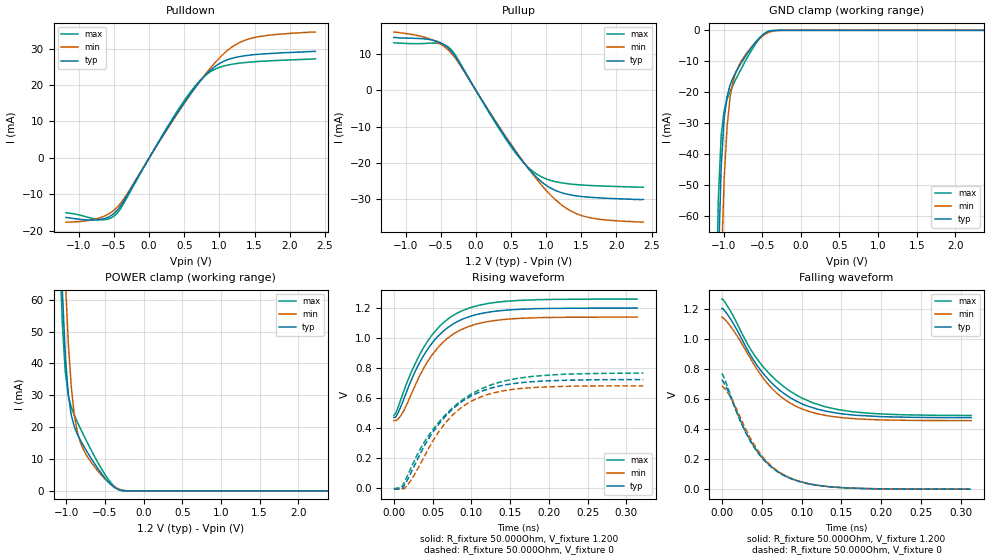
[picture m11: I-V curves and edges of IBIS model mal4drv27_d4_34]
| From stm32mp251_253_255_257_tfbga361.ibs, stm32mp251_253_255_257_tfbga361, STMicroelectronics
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[Model] mal4drv27_d4_34
Model_type   I/O
Polarity   Non-Inverting
Enable   Active-High
C_comp   1.656pF   1.652pF   1.661pF
C_comp_pullup   829.373fF   822.555fF   836.725fF
C_comp_pulldown 737.416fF   735.607fF   748.448fF
Vinh = 852.000mV
Vinl = 737.000mV
Vmeas = 795.000mV
Vref = 1.200V
Rref = 50Ohms
Cref = 0pF
[Model Spec]
Vinh   852.000mV   812.000mV   892.000mV
Vinl   737.000mV   697.000mV   777.000mV
Vmeas   795.000mV   755.000mV   834.000mV
Vref   1.200V   1.140V   1.260V
D_overshoot_ampl_h 0.24 NA   NA
D_overshoot_ampl_l 0.24 NA   NA
D_overshoot_area_l 300.000m NA   NA
D_overshoot_area_h 300.000m NA   NA
[Receiver Thresholds]
Vth = 795.000mV
Vth_min = 755.000mV
Vth_max = 834.000mV
Vinh_ac = 68.000mV
Vinh_dc = 68.000mV
Vinl_ac = -68.000mV
Vinl_dc = -68.000mV
Tslew_ac = 5.000ns
Threshold_sensitivity = 0.5
Reference_supply Pullup_ref
[Temperature Range]   25.000   125.000   -40.000
[Voltage Range]   1.200V   1.140V   1.260V
[GND Clamp Reference]   0.00V   0.00V   0.00V
[C Comp Corner]
| variable   typ   min   max
C_comp 1.661pF   1.656pF   1.652pF
C_comp_pullup 829.373fF   836.725fF   822.555fF
C_comp_pulldown 735.607fF   748.448fF   737.416fF
[Pulldown Reference]   0.00V   0.00V   0.00V
[POWER Clamp Reference]   1.200V   1.140V   1.260V
[Pullup Reference]   1.200V   1.140V   1.260V
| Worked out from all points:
|   slope of the pulldown table from 0 to 0.18 V, typ, clamps not added: 31.5 ohm
|   slope of the pullup table from 0 to 0.18 V, typ, clamps not added: 31.8 ohm
|   GND clamp passes 1 mA (typ) near -0.47 V on its own axis
|   POWER clamp passes 1 mA (typ) near -0.37 V on its own axis
|   rising waveform, R_fixture 50.000Ohm, V_fixture 1.200: 20-80 % time 51.2ps typ, 50.7ps min, 52.2ps max; typ from 0.472 V to 1.2 V
|   rising waveform, R_fixture 50.000Ohm, V_fixture 0: 20-80 % time 62.5ps typ, 57.9ps min, 71.8ps max; typ from -0.006 V to 0.724 V
|   falling waveform, R_fixture 50.000Ohm, V_fixture 1.200: 20-80 % time 62.9ps typ, 58.9ps min, 69.2ps max; typ from 1.2 V to 0.475 V
|   falling waveform, R_fixture 50.000Ohm, V_fixture 0: 20-80 % time 49.1ps typ, 48.9ps min, 49.5ps max; typ from 0.727 V to 0 V
[GND Clamp]
-1.184V   -313.6mA   -372.3mA   -285.9mA
-1.107V   -133mA     -190.9mA   -103.4mA
-1.069V   -76.66mA   -125mA     -55.43mA
-1.031V   -44.19mA   -77.99mA   -34.02mA
-992.7mV  -28.51mA   -48.19mA   -25.88mA
-954.6mV  -21.35mA   -31.1mA    -22.21mA
-916.4mV  -17.7mA    -21.78mA   -19.79mA
-878.2mV  -15.35mA   -16.61mA   -17.73mA
-801.8mV  -11.82mA   -11.34mA   -13.9mA
-610.9mV  -4.628mA   -4.618mA   -5.371mA
-458.2mV  -822.8uA   -1.198mA   -809uA
2.367V    18.95nA    454.6nA    6.243nA
[Power Clamp]
-1.167V   171.5mA    206.4mA    156.1mA
-1.091V   92.44mA    126.6mA    77.99mA
-1.053V   63.02mA    93.75mA    52.4mA
-1.015V   42.49mA    66.9mA     37.37mA
-976.4mV  30.34mA    46.72mA    30.02mA
-938.2mV  23.88mA    32.9mA     26.3mA
-900mV    20.31mA    24.15mA    23.84mA
-823.6mV  16.11mA    15.49mA    19.79mA
-747.3mV  12.87mA    11.46mA    16.02mA
-518.2mV  4.545mA    4.187mA    5.836mA
-365.4mV  856.5uA    1.078mA    1.107mA
2.384V    -12.74nA   -415.5nA   -4.625nA
[Pulldown]
-1.184V   -16.3mA    -17.6mA    -15mA
-725.5mV  -16.94mA   -16.55mA   -16.87mA
-572.7mV  -16.13mA   -15.3mA    -16.68mA
-458.2mV  -14.43mA   -13.55mA   -15.2mA
-305.5mV  -9.986mA   -9.58mA    -10.51mA
420mV     12.95mA    12.68mA    13.44mA
687.3mV   20.12mA    20.08mA    20.48mA
878.2mV   24.14mA    24.8mA     23.72mA
1.145V    27.12mA    29.93mA    25.57mA
1.375V    28.05mA    32.33mA    26.17mA
1.756V    28.67mA    33.75mA    26.66mA
2.367V    29.2mA     34.5mA     27.18mA
[Pullup]
-1.167V   14.6mA     16.1mA     13.16mA
-594.5mV  13.79mA    13.71mA    13.07mA
-480mV    12.94mA    12.49mA    12.8mA
-365.4mV  11.21mA    10.59mA    11.52mA
-250.9mV  8.092mA    7.721mA    8.443mA
283.6mV   -8.835mA   -8.586mA   -9.154mA
550.9mV   -16.57mA   -16.29mA   -16.91mA
780mV     -22.29mA   -22.41mA   -21.87mA
1.009V    -26.32mA   -27.79mA   -24.51mA
1.276V    -28.56mA   -32.42mA   -25.69mA
1.505V    -29.32mA   -34.57mA   -26.12mA
2.384V    -30.1mA    -36.4mA    -26.74mA
[Ramp]
R_load=50.000Ohm
dV/dt_r   434.850mV/58.000ps  410.159mV/55.500ps  461.550mV/63.000ps
dV/dt_f   434.850mV/57.000ps  410.159mV/55.000ps  461.550mV/61.000ps
[Rising waveform]
R_fixture=50.000Ohm
V_fixture=1.200
V_fixture_min=1.140
V_fixture_max=1.260
0s        472.2mV    451.1mV    485.7mV
4ps       488.5mV    455.5mV    521.4mV
12ps      584.3mV    509.5mV    637.6mV
27ps      773.4mV    680.4mV    825.2mV
41ps      906.4mV    822.7mV    959.8mV
62ps      1.038V     965.3mV    1.094V
85ps      1.118V     1.051V     1.175V
113ps     1.164V     1.102V     1.222V
153ps     1.189V     1.129V     1.248V
314ps     1.2V       1.14V      1.26V
[Rising waveform]
R_fixture=50.000Ohm
V_fixture=0
0s        -6.059mV   -4.191mV   -2.794mV
10ps      -6.059mV   -4.191mV   6.233mV
19ps      70.79mV    30.63mV    100.5mV
38ps      270mV      200.4mV    297.1mV
59ps      434.2mV    384.6mV    446.5mV
82ps      554.7mV    516.6mV    563mV
108ps     635.5mV    599.6mV    649.9mV
140ps     684.9mV    647.8mV    711.4mV
178ps     709.4mV    670.3mV    744.9mV
322ps     723.8mV    682.3mV    766.6mV
[Falling waveform]
R_fixture=50.000Ohm
V_fixture=1.200
V_fixture_min=1.140
V_fixture_max=1.260
0s        1.201V     1.143V     1.263V
14ps      1.104V     1.06V      1.154V
33ps      917mV      893.8mV    956.7mV
50ps      781mV      750.8mV    825mV
62ps      708.4mV    673.6mV    754.6mV
75ps      647.2mV    610.5mV    692.4mV
99ps      570.8mV    536.7mV    609mV
130ps     518.6mV    489.8mV    547.1mV
166ps     492mV      468mV      513.3mV
313ps     475mV      455.5mV    489.5mV
[Falling waveform]
R_fixture=50.000Ohm
V_fixture=0
0s        727.1mV    685.8mV    769.7mV
11ps      612.1mV    611.4mV    624.1mV
26ps      419.1mV    443.8mV    424.4mV
40ps      281.7mV    300mV      285.9mV
50ps      209.9mV    222.7mV    213.6mV
61ps      151.4mV    159.2mV    154.3mV
83ps      77.42mV    80.93mV    79.63mV
112ps     32.15mV    32.66mV    33.46mV
150ps     9.76mV     9.955mV    10.61mV
312ps     61.98uV    67.76uV    72.04uV
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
